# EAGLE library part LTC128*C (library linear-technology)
3V Micropower Sampling 12-Bit A/D Converters Source: http://www.linear.com/pc/downloadDocument.do?navId=H0,C1,C1155,C1001,C1158,P1489,D3463
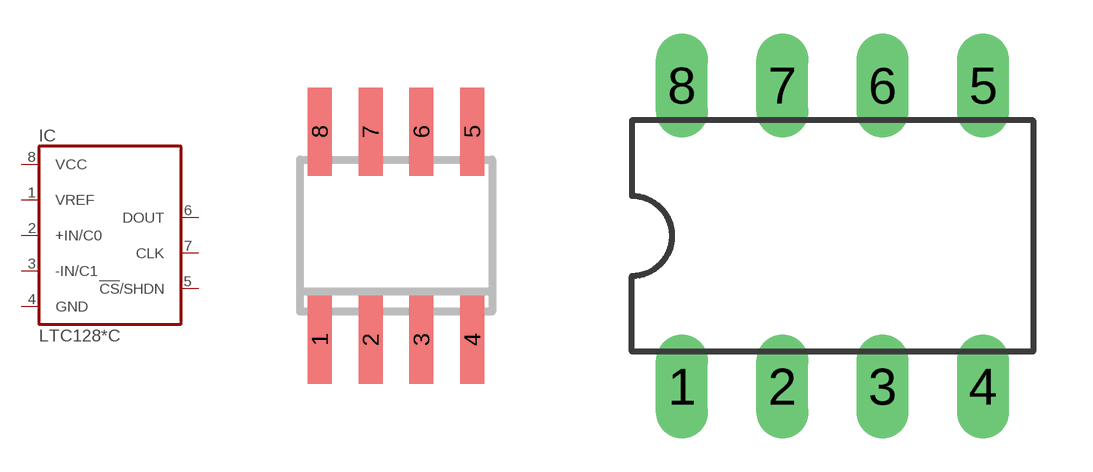
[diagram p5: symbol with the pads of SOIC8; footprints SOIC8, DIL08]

Designator prefix IC

## LTC1285CS8 (MPN: LTC1285CS8; OC_FARNELL: 4767585; OC_NEWARK: 56M0033), LTC1288CS8 (MPN: LTC1288CS8; OC_FARNELL: 9561013; OC_NEWARK: 56M0059)  [SOIC8]
1  VREF  in
2  +IN/C0  in
3  -IN/C1  in
4  GND  pwr
5  !CS!/SHDN  out
6  DOUT  out
7  CLK  in
8  VCC  pwr

## LTC1285CN8 (MPN: LTC1285CN8; OC_FARNELL: 1330820; OC_NEWARK: 56M0031), LTC1288CN8 (MPN: LTC1288CN8; OC_FARNELL: 1330821; OC_NEWARK: 56M0057)  [DIL08]
Pads as for SOIC8

## Footprint SOIC8 (pad centres in mm)
Small Outline IC
smd 0.6 x 2.2: 1 -1.905,-2.6; 2 -0.635,-2.6; 3 0.635,-2.6; 4 1.905,-2.6; 5 1.905,2.6; 6 0.635,2.6; 7 -0.635,2.6; 8 -1.905,2.6

## Footprint DIL08 (pad centres in mm)
Dual In Line Package
drill 0.813 long: 1 -3.81,-3.81; 2 -1.27,-3.81; 3 1.27,-3.81; 4 3.81,-3.81; 5 3.81,3.81; 6 1.27,3.81; 7 -1.27,3.81; 8 -3.81,3.81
